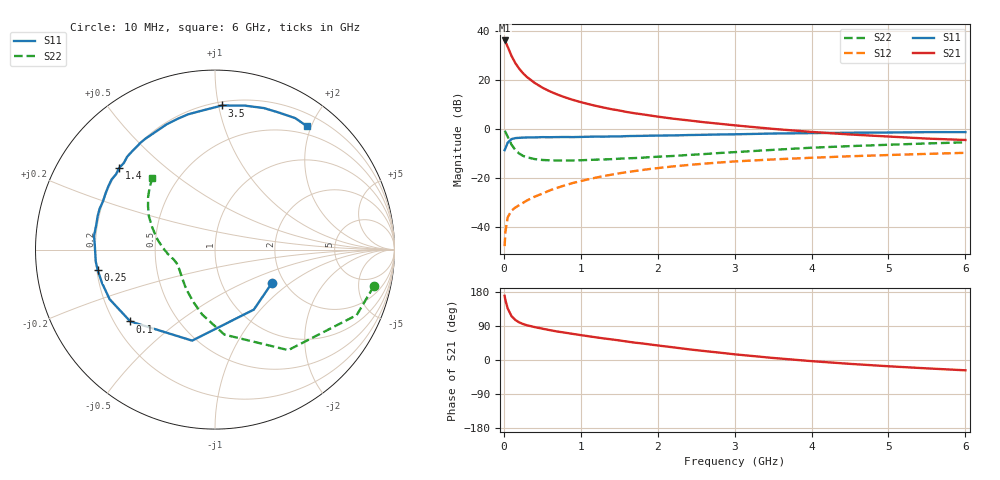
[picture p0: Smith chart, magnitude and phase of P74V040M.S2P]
! SIEMENS Small Signal Semiconductors
! BFP196
! Si NPN RF Bipolar Junction Transistor in SOT143
! VCE = 4 V  IC = 40 mA
! Common Emitter S-Parameters:  May  1996
# GHz  S  MA  R  50
!  f  S11  S21  S12  S22
! GHz  MAG  ANG  MAG  ANG  MAG  ANG  MAG  ANG
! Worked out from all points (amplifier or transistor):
!   36 points, 10 MHz to 6 GHz, reference 50 ohm
!   highest |S21| = 36.2 dB at 10 MHz (marker M1)
!   |S21| within 3 dB of that: start of sweep to 55.7 MHz
!   unconditionally stable (mu >= 1): 497.7 MHz to 4.195 GHz
!   at 250 MHz: K = 0.78, MSG = 26.5 dB, |S12| = -30.2 dB
!   at 1.4 GHz: K = 1.09, MAG = 11.6 dB, |S12| = -18.7 dB
!   at 6 GHz: K = 0.97, MSG = 2.6 dB, |S12| = -9.8 dB
!   S11 on the Smith chart (normalised r, x): 10 MHz: 1.71, -0.75; 100 MHz: 0.27, -0.34; 250 MHz: 0.20, -0.08; 1.4 GHz: 0.20, +0.36; 3.5 GHz: 0.23, +1.02; 6 GHz: 0.37, +1.94
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0.01  0.3675 -30.9  64.27 169.4  0.004 80.6  0.9085 -12.9
0.02  0.3983 -57.1  60.62 158.6  0.0078 74.6  0.8697 -24.8
0.05  0.5229 -104.1  47.8 136.0  0.0155 55.8  0.6931 -53.9
0.1  0.6187 -139.7  30.99 115.6  0.0214 47.7  0.4765 -83.7
0.15  0.6487 -154.7  22.05 105.5  0.0247 46.7  0.369 -101.1
0.2  0.6566 -163.6  17 99.2  0.0276 48.2  0.3134 -113.1
0.25  0.6634 -170.0  13.69 94.9  0.0308 50.6  0.2803 -122.7
0.3  0.6677 -174.3  11.5 91.7  0.0343 53.1  0.2632 -129.3
0.4  0.6696 178.4  8.73 86.9  0.0411 56.5  0.2414 -139.4
0.5  0.6783 173.6  6.983 82.7  0.0474 58.6  0.2315 -146.3
0.6  0.6757 168.4  5.835 78.7  0.0555 59.7  0.2275 -151.1
0.7  0.68 164.1  5.015 75.0  0.0629 60.1  0.2262 -154.6
0.9  0.6795 156.8  3.907 68.8  0.0785 59.7  0.2263 -160.0
1.1  0.6909 149.4  3.213 62.7  0.0932 58.6  0.2315 -163.6
1.4  0.7019 139.4  2.526 54.4  0.1158 55.6  0.2405 -168.0
1.7  0.7166 130.0  2.087 45.9  0.1374 51.8  0.2533 -172.5
2.2  0.7351 116.6  1.618 33.5  0.1709 45.0  0.2794 -179.3
2.8  0.7684 101.3  1.275 19.5  0.2054 36.6  0.3211 170.9
3.5  0.8039 87.2  1 5.4  0.2375 26.9  0.3726 160.2
4.5  0.8343 70.9  0.768 -10.2  0.2756 15.1  0.4444 147.1
5.5  0.858 58.6  0.634 -22.1  0.3083 4.4  0.5036 136.3
6  0.8577 53.3  0.593 -27.2  0.3241 -1.4  0.5308 131.0
